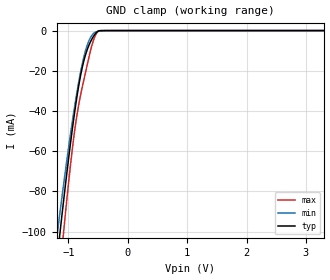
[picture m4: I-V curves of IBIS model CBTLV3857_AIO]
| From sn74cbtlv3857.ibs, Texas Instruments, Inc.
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[Model]   CBTLV3857_AIO
Model_type  Terminator
| variable   typ   min   max
C_comp   3.12pF   2.59pF   3.57pF
| C_tri-state   3.12pF   2.59pF   3.57pF
[Temperature Range]   40   100   -40
| Ambient temperature   25   85   -40
[Voltage range]   3.3   3   3.6
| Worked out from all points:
|   GND clamp passes 1 mA (typ) near -0.53 V on its own axis
[GND Clamp]
| CBTLV3857_AIO
|   Voltage   I(typ)   I(min)   I(max)
-3.3V     -768.7mA   -675.1mA   -909.5mA
-1.19V    -113.6mA   -101.8mA   -134.6mA
-1.135V   -98.8mA    -88.91mA   -117.1mA
-1.085V   -85.71mA   -77.48mA   -101.5mA
-920mV    -45.97mA   -42.54mA   -55.6mA
-860mV    -33.63mA   -31.37mA   -42.79mA
-800mV    -23.16mA   -21.45mA   -32.82mA
-735mV    -14.48mA   -12.59mA   -23.88mA
-670mV    -8.454mA   -6.204mA   -15.34mA
-545mV    -1.518mA   -769.9uA   -2.363mA
-440mV    -18.4uA    -153.5uA   -5.93uA
3.3V      1.225nA    60.97nA    15.21pA
